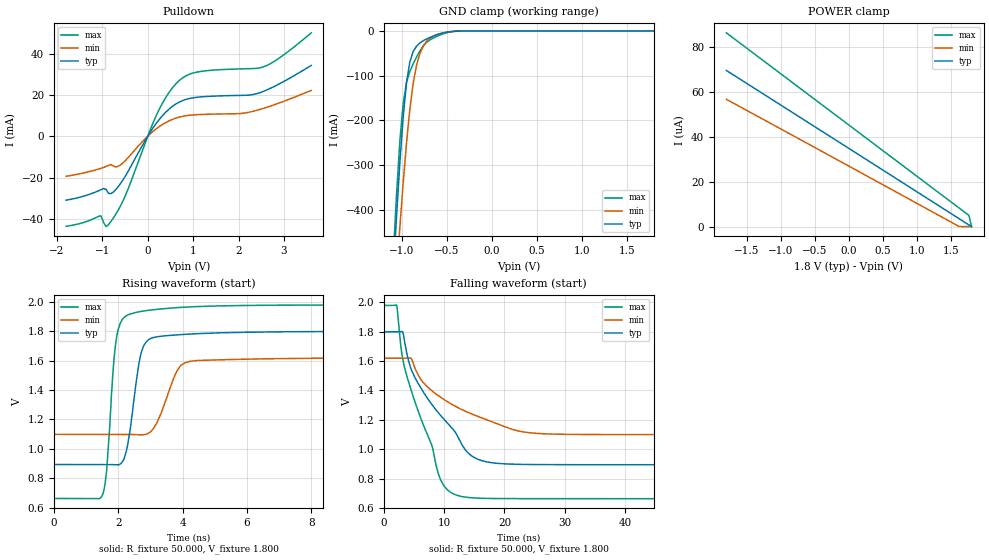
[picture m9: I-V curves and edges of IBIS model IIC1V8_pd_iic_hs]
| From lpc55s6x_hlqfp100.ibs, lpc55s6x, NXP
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|   Model IIC1V8_pd_iic_hs
[Model] IIC1V8_pd_iic_hs
Model_type I/O_open_drain
Polarity   Non-Inverting
Enable   Active-Low
Vinl =  0.540V
Vinh =  1.260V
Vmeas =  0.900V
Cref =  0.0F
Rref =  100.000
Vref =  1.800V
C_comp   2.439pF   2.391pF   2.494pF
C_comp_pulldown   1.725pF   1.661pF   1.781pF
C_comp_power_clamp   0.386pF   0.354pF   0.433pF
[Model Spec]
Vinh   1.260V   1.134V   1.386V
Vinl   0.540V   0.486V   0.594V
Vmeas   0.900V   0.810V   0.990V
Vref   1.800V   1.620V   1.980V
Cref   0.0F   0.0F   0.0F
Rref   100.000   100.000   100.000
[Temperature Range]   25.000   0.125k   -40.000
[Voltage Range]   1.800V   1.620V   1.980V
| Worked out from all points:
|   slope of the pulldown table from 0 to 0.27 V, typ, clamps not added: 31.5 ohm
|   GND clamp passes 1 mA (typ) near -0.44 V on its own axis
|   rising waveform, R_fixture 50.000, V_fixture 1.800: 20-80 % time 346ps typ, 537ps min, 256ps max; typ from 0.894 V to 1.8 V
|   falling waveform, R_fixture 50.000, V_fixture 1.800: 20-80 % time 8.41ns typ, 11.3ns min, 5.72ns max; typ from 1.8 V to 0.894 V
[Pulldown]
|Voltage   I(typ)   I(min)   I(max)
-1.8V     -30.97mA   -19.41mA   -43.61mA
-1.03V    -25.91mA   -15.56mA   -38.59mA
-920mV    -25.75mA   -14.67mA   -43.75mA
-865mV    -27.69mA   -14.16mA   -42.79mA
-700mV    -25.69mA   -14.87mA   -37.58mA
-480mV    -18.8mA    -11.48mA   -28.03mA
235mV     7.619mA    4.356mA    12.23mA
455mV     12.83mA    7.267mA    20.76mA
730mV     16.88mA    9.427mA    27.6mA
1.17V     19mA       10.49mA    31.33mA
2.545V    21.66mA    13.44mA    33.54mA
3.6V      34.22mA    22.14mA    50.01mA
[GND_clamp]
|Voltage   I(typ)   I(min)   I(max)
-1.8V     -3.488A    -3.23A     -3.872A
-1.097V   -545.5mA   -658.5mA   -507mA
-1.06V    -414.6mA   -546.1mA   -365mA
-1.023V   -294.9mA   -439.1mA   -245.9mA
-986mV    -192.4mA   -339.6mA   -162mA
-949mV    -115.6mA   -250.3mA   -115.1mA
-912mV    -69.19mA   -175.2mA   -90.62mA
-838mV    -34.02mA   -77.16mA   -58.5mA
-764mV    -21.82mA   -34.11mA   -33.6mA
-653mV    -11.43mA   -11.65mA   -15.83mA
-431mV    -835.3uA   -879.6uA   -1.141mA
1.8V      0A         0A         0A
[POWER_clamp]
|Voltage   I(typ)   I(min)   I(max)
-1.8V     69.55uA    56.68uA    86.29uA
1.615V    3.579uA    80.87nA    8.337uA
1.763V    715.6nA    0A         4.957uA
1.8V      0A         0A         0A
[Ramp]
| variable   typ   min   max
dV/dt_r   0.543/0.347n   0.312/0.537n   0.789/0.254n
dV/dt_f   0.543/8.400n   0.312/11.331n   0.789/5.717n
R_load = 50.000
[Rising Waveform]
R_fixture= 50.000
V_fixture= 1.800
V_fixture_min= 1.620
V_fixture_max= 1.980
|time   V(typ)   V(min)   V(max)
0s        893.8mV    1.098V     663mV
1.52ns    893.8mV    1.098V     691.5mV
1.64ns    893.9mV    1.098V     849.9mV
1.9ns     891.9mV    1.098V     1.676V
2.15ns    918.8mV    1.099V     1.885V
2.65ns    1.587V     1.096V     1.931V
2.84ns    1.718V     1.097V     1.938V
3.94ns    1.776V     1.565V     1.961V
5.03ns    1.787V     1.604V     1.97V
250ns     1.798V     1.619V     1.978V
[Falling Waveform]
R_fixture= 50.000
V_fixture= 1.800
V_fixture_min= 1.620
V_fixture_max= 1.980
|time   V(typ)   V(min)   V(max)
0s        1.798V     1.619V     1.978V
2.12ns    1.798V     1.619V     1.978V
2.94ns    1.801V     1.619V     1.657V
3.51ns    1.714V     1.618V     1.54V
5.11ns    1.49V      1.555V     1.327V
9.34ns    1.232V     1.355V     798.3mV
13.58ns   992.2mV    1.257V     673.3mV
17.68ns   909.1mV    1.191V     664.6mV
29.96ns   894.5mV    1.101V     663.2mV
250ns     893.8mV    1.098V     663.1mV
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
